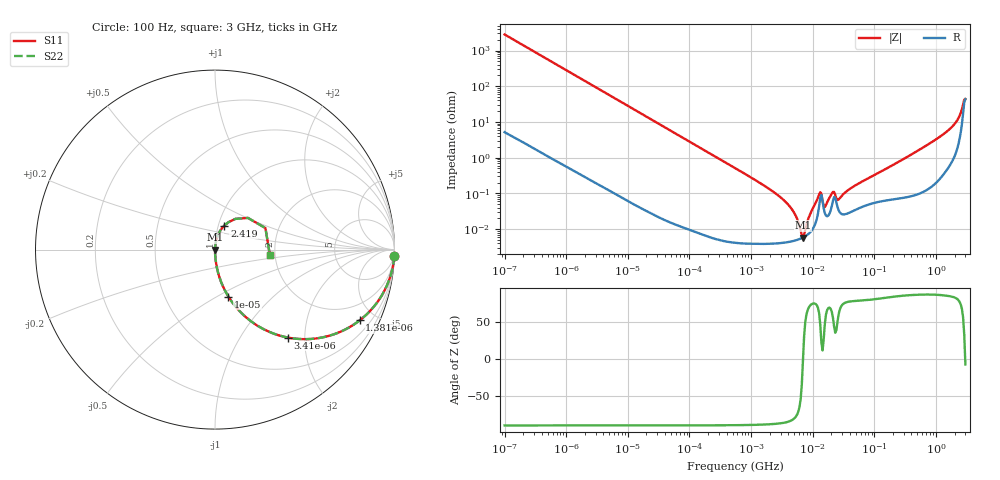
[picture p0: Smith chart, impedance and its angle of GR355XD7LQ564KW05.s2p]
!Murata Part Number: GR355XD7LQ564KW05
!These Parameters are Measured in Series Mode Connection
!Data Generated on Jun 10, 2025
!  o--ll--o
!Port1  Port2
!  o------o
!Operation Temp=25[degC], DC Bias Voltage=0[V]
!Freq. Start=100[Hz] Stop=3[GHz] 401[Steps]
# Hz S RI R 50
!Freq.(Hz) S11(Real) S11(Imag) S21(Real) S21(Imag) S12(Real) S12(Imag) S22(Real) S22(Imag)
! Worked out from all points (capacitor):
!   401 points, 100 Hz to 3 GHz, reference 50 ohm
!   read as one part in series: C = 566 nF near 109 Hz
!   lowest |Z| = 5.83 mohm at 6.941 MHz (marker M1)
!   series resonance near 6.954 MHz, so ESL is about 930 pH
!   S11 on the Smith chart (normalised r, x): 100 Hz: 1, -56; 1.381 kHz: 1.01, -4.09; 3.41 kHz: 1.00, -1.66; 10 kHz: 1.00, -0.57; 2.419 GHz: 1.07, +0.29; 3 GHz: 1.87, -0.12
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100  0.9987 -0.0355  0.00133 0.0355  0.00133 0.0355  0.9987 -0.0355
559  0.9618 -0.1908  0.0382 0.1908  0.0382 0.1908  0.9618 -0.1908
1381  0.8063 -0.3942  0.1937 0.3942  0.1937 0.3942  0.8063 -0.3942
1788  0.7133 -0.4512  0.2867 0.4512  0.2867 0.4512  0.7133 -0.4512
3410  0.4073 -0.4903  0.5927 0.4903  0.5927 0.4903  0.4073 -0.4903
10003  0.0746 -0.2617  0.9254 0.2617  0.9254 0.2617  0.0746 -0.2617
31977  0.008 -0.0879  0.992 0.0879  0.992 0.0879  0.008 -0.0879
547723  6.82e-05 -0.00516  0.9999 0.00516  0.9999 0.00516  6.82e-05 -0.00516
3339322  4.21e-05 -0.000663  1 0.000663  1 0.000663  4.21e-05 -0.000663
4711951  4.62e-05 -0.000335  1 0.000335  1 0.000335  4.62e-05 -0.000335
6941223  5.83e-05 -1.6e-06  0.9999 1.6e-06  0.9999 1.6e-06  5.83e-05 -1.6e-06
9794414  9.6e-05 0.000338  0.9999 -0.000338  0.9999 -0.000338  9.6e-05 0.000338
1.268047e7  0.000434 0.000811  0.9996 -0.000811  0.9996 -0.000811  0.000434 0.000811
1.641694e7  0.00024 0.000416  0.9998 -0.000416  0.9998 -0.000416  0.00024 0.000416
2.035898e7  0.00044 0.000888  0.9996 -0.000888  0.9996 -0.000888  0.00044 0.000888
2.635803e7  0.000337 0.000591  0.9997 -0.000591  0.9997 -0.000591  0.000337 0.000591
4.612319e7  0.000331 0.00154  0.9997 -0.00154  0.9997 -0.00154  0.000331 0.00154
1.751444e8  0.000686 0.00546  0.9993 -0.00546  0.9993 -0.00546  0.000686 0.00546
1.268426e9  0.00493 0.0429  0.9951 -0.0429  0.9951 -0.0429  0.00493 0.0429
1.868531e9  0.014 0.0744  0.986 -0.0744  0.986 -0.0744  0.014 0.0744
2.419119e9  0.052 0.134  0.948 -0.134  0.948 -0.134  0.052 0.134
3e9  0.3052 -0.0281  0.6948 0.0281  0.6948 0.0281  0.3052 -0.0281
